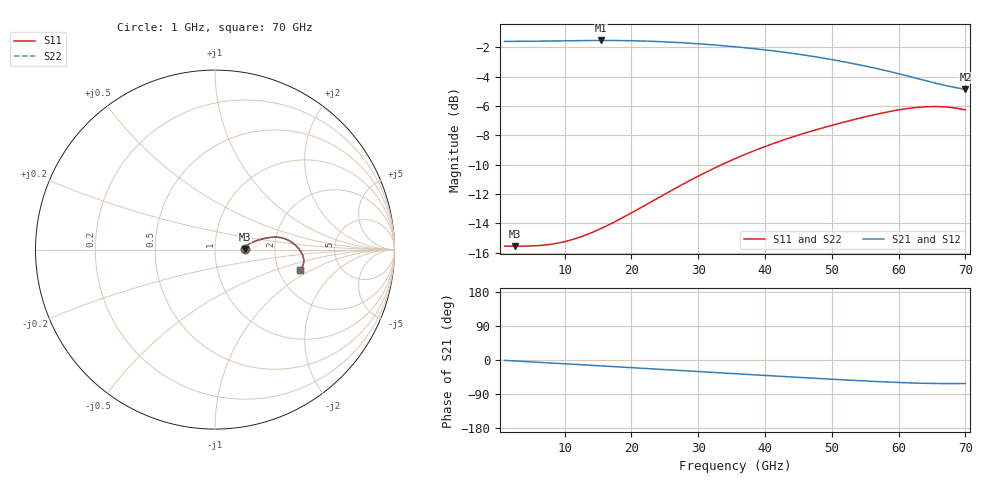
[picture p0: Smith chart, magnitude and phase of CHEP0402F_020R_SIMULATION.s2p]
! Touchstone file exported from HFSS 2026.1.0
!  File:  S:/COMPOSANTS_3D_CRYPTES/CHEP0402F/2026R1/PCB_&_COMP/PCB_V1.1.003_CHEP0402F_V1.aedt
!  $RV = 20ohm
# GHz S MA R 50.000000
! Terminal data exported
! Port[1] = LINE_T1
! Port[2] = LINE_T2
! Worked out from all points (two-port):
!   401 points, 1 GHz to 70 GHz, reference 50 ohm
!   highest |S21| = -1.52 dB at 15.49 GHz (marker M1); lowest = -4.9 dB at 70 GHz (marker M2)
!   |S21| within 3 dB of the highest: start of sweep to 66.31 GHz
!   lowest |S11| = -15.6 dB at 2.553 GHz (marker M3), VSWR 1.40, Z = 70 + j0.399 ohm
!   |S11| at or under -10 dB: start of sweep to 33.49 GHz
!   |S22| runs from -15.6 to -6.0 dB; largest |S21 - S12| = 3.5e-14
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1  0.1669 0.3  0.8332 -1.0  0.8332 -1.0  0.1669 0.3
2.5525  0.1668 1.0  0.8336 -2.6  0.8336 -2.6  0.1667 0.9
5.6575  0.1673 2.6  0.8345 -5.6  0.8345 -5.6  0.1672 2.7
7.9  0.1692 4.2  0.8359 -7.8  0.8359 -7.8  0.1691 4.2
10.1425  0.1731 5.8  0.8374 -10.1  0.8374 -10.1  0.1729 5.9
12.5575  0.1799 7.6  0.8387 -12.5  0.8387 -12.5  0.1797 7.6
15.49  0.1917 9.4  0.8394 -15.6  0.8394 -15.6  0.1915 9.5
19.8025  0.2154 11.3  0.8376 -20.1  0.8376 -20.1  0.2151 11.4
24.115  0.2446 12.3  0.832 -24.6  0.832 -24.6  0.2444 12.4
29.8075  0.2877 12.7  0.8185 -30.4  0.8185 -30.4  0.2876 12.7
35.5  0.3316 12.0  0.7988 -36.2  0.7988 -36.2  0.3316 12.0
41.5375  0.3756 10.1  0.772 -42.3  0.772 -42.3  0.3757 10.1
44.2975  0.3944 8.8  0.7575 -45.1  0.7575 -45.1  0.3945 8.8
47.0575  0.4124 7.2  0.7413 -47.9  0.7413 -47.9  0.4125 7.2
49.99  0.4308 5.3  0.7224 -50.7  0.7224 -50.7  0.4309 5.3
52.9225  0.4487 3.1  0.7019 -53.5  0.7019 -53.5  0.4487 3.2
55.855  0.4657 0.8  0.6801 -56.1  0.6801 -56.1  0.4657 0.8
58.615  0.4802 -1.7  0.658 -58.4  0.658 -58.4  0.4802 -1.7
61.8925  0.4936 -4.9  0.6301 -60.6  0.6301 -60.6  0.4936 -4.8
64.6525  0.4992 -7.7  0.6068 -61.8  0.6068 -61.8  0.4992 -7.7
67.24  0.4974 -10.5  0.5878 -62.2  0.5878 -62.2  0.4976 -10.4
70  0.4865 -13.3  0.5715 -62.0  0.5715 -62.0  0.4866 -13.2
